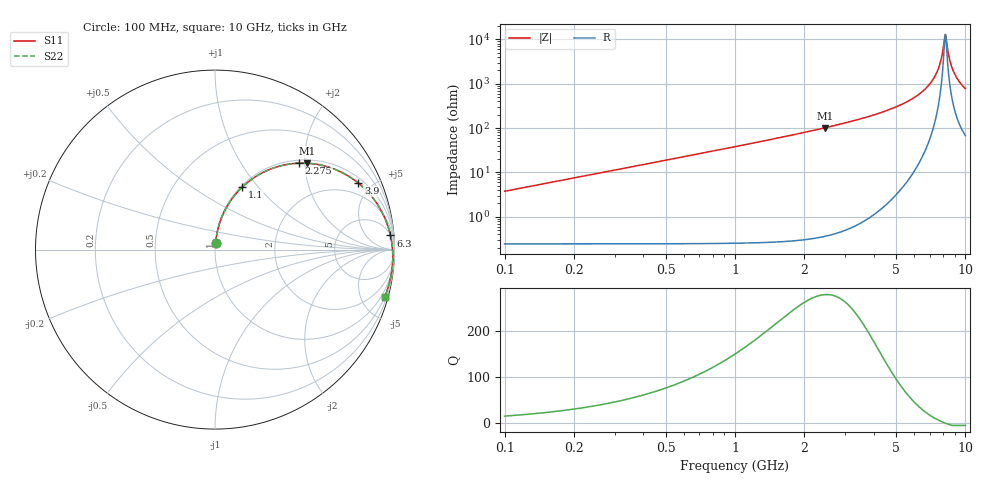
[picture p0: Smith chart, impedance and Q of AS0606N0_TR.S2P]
!AVX Corporation
! PN: AS0606N0*TR
! DESCRIPTION: SQUARE AIR CORE INDUCTOR, 6.0nH, 3 Turns
# MHZ S MA R 50
!Freq  MagS11  AngS11  MagS21  AngS21  MagS12  AngS12  MagS22  AngS22
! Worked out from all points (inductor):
!   397 points, 100 MHz to 10 GHz, reference 50 ohm
!   read as one part in series: L = 5.98 nH near 125 MHz
!   highest Q = 280 at 2.45 GHz (marker M1), where L = 6.57 nH
!   self-resonance near 8.175 GHz
!   S11 on the Smith chart (normalised r, x): 100 MHz: 1.00, +0.07; 1.1 GHz: 1.02, +0.83; 2.275 GHz: 1.07, +1.87; 3.9 GHz: 1.26, +4.16; 6.3 GHz: 6, +23; 10 GHz: 0.50, -7.22
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100  0.03685 84.0  0.9969 -2.2  0.9969 -2.2  0.03686 84.0
225  0.08259 83.4  0.9941 -4.9  0.9941 -4.9  0.08261 83.4
425  0.1549 79.9  0.9855 -9.2  0.9855 -9.2  0.1549 79.9
700  0.2512 74.4  0.9655 -15.1  0.9655 -15.1  0.2512 74.4
1100  0.3812 66.4  0.9221 -23.3  0.9221 -23.3  0.3812 66.4
1750  0.5596 54.4  0.8264 -35.4  0.8264 -35.4  0.5597 54.4
2275  0.6723 45.8  0.7377 -44.0  0.7377 -44.0  0.6725 45.8
2450  0.7041 43.1  0.7075 -46.7  0.7075 -46.7  0.7042 43.1
3400  0.8343 30.5  0.5476 -59.2  0.5476 -59.2  0.8344 30.5
3900  0.8802 24.9  0.4697 -64.8  0.4697 -64.8  0.8803 24.9
5050  0.9469 14.1  0.3112 -75.3  0.3112 -75.3  0.947 14.1
6300  0.9807 4.6  0.169 -83.7  0.169 -83.7  0.9809 4.6
6700  0.9862 2.0  0.1291 -85.7  0.1291 -85.7  0.9864 2.0
7250  0.9907 -1.5  0.07821 -87.0  0.07821 -87.0  0.9909 -1.5
7650  0.9922 -3.8  0.04391 -85.0  0.04391 -85.0  0.9924 -3.8
7900  0.9925 -5.2  0.02388 -77.8  0.02388 -77.8  0.9927 -5.2
8175  0.9923 -6.7  0.007664 -13.9  0.007664 -13.9  0.9925 -6.7
8225  0.9922 -7.0  0.008221 13.8  0.008221 13.8  0.9924 -7.0
8350  0.9919 -7.7  0.01477 50.0  0.01477 50.0  0.9921 -7.7
8575  0.9912 -8.8  0.03044 65.4  0.03044 65.4  0.9914 -8.8
8900  0.9897 -10.5  0.05339 70.0  0.05339 70.0  0.9898 -10.5
10000  0.9813 -15.7  0.1249 69.3  0.1249 69.3  0.9815 -15.7
